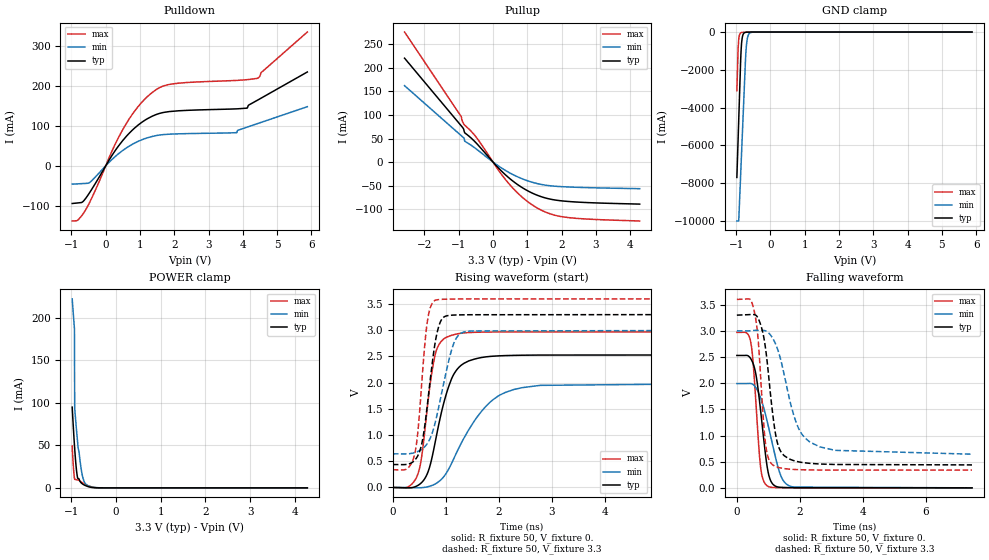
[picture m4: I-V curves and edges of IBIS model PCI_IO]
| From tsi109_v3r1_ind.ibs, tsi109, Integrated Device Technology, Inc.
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|   MODEL PCI_IO
[Model]   PCI_IO
Model_type  I/O
C_comp 4.536p 4.202p 4.874p
Polarity   Non-Inverting
Enable   Active-High
Vinl =   0.80V
Vinh =   2.00V
Vmeas =   1.50V
Cref =   10pF
Rref =   50
Vref=   0.0V
[Model Spec]
[Temperature Range]   27.0   125.0   -40.0
[Voltage Range] 3.3 3. 3.6
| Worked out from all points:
|   slope of the pulldown table from 0 to 0.495 V, typ, clamps not added: 7.81 ohm
|   slope of the pullup table from 0 to 0.495 V, typ, clamps not added: 13.9 ohm
|   GND clamp passes 1 mA (typ) near -0.58 V on its own axis
|   POWER clamp passes 1 mA (typ) near -0.59 V on its own axis
|   rising waveform, R_fixture 50, V_fixture 0.: 20-80 % time 365ps typ, 723ps min, 222ps max; typ from 0 V to 2.53 V
|   rising waveform, R_fixture 50, V_fixture 3.3: 20-80 % time 214ps typ, 317ps min, 159ps max; typ from 0.438 V to 3.3 V
|   falling waveform, R_fixture 50, V_fixture 0.: 20-80 % time 295ps typ, 484ps min, 203ps max; typ from 2.53 V to 0 V
|   falling waveform, R_fixture 50, V_fixture 3.3: 20-80 % time 338ps typ, 623ps min, 226ps max; typ from 3.3 V to 0.438 V
[Pulldown]
-976.9mV  -94.66mA   -46.06mA   -138.7mA
-817.5mV  -93.23mA   -45.29mA   -136.5mA
-595.7mV  -83.14mA   -44.21mA   -112.2mA
-429.3mV  -61.97mA   -39.17mA   -84.92mA
492.7mV   63.11mA    38.33mA    90.31mA
936.3mV   101.8mA    61.1mA     147.9mA
1.352V    124.6mA    73.73mA    184.1mA
1.851V    136.3mA    79.48mA    204.5mA
3.82V     143.1mA    83.35mA    214.6mA
4.125V    144.9mA    97.25mA    216.4mA
4.43V     165.1mA    106.2mA    220mA
5.879V    235.8mA    148.6mA    336.1mA
[Pullup]
-2.579V   220.8mA    162.3mA    276.3mA
-929mV    77.21mA    56.24mA    96.97mA
-887.4mV  73.58mA    53.57mA    85.73mA
-838.9mV  65.18mA    49.35mA    79.56mA
-818.1mV  61.78mA    43.99mA    77.84mA
-471.5mV  38.99mA    26.83mA    51.07mA
277.2mV   -21.28mA   -14.01mA   -29.14mA
623.8mV   -42.97mA   -28.22mA   -58.92mA
942.6mV   -58.4mA    -38.19mA   -80.33mA
1.442V    -74.52mA   -48.11mA   -103.5mA
1.969V    -82.31mA   -52.22mA   -115.7mA
4.277V    -89.5mA    -56.68mA   -125.4mA
[GND Clamp]
-976.9mV  -7.694A    -10A       -3.11A
-940.4mV  -5.645A    -10A       -848.5mA
-923.3mV  -4.682A    -10A       -400.9mA
-899.6mV  -3.359A    -8.991A    -148.3mA
-863.2mV  -1.353A    -7.407A    -43.18mA
-837.4mV  -553.5mA   -6.29A     -25.04mA
-794.5mV  -126.9mA   -4.431A    -15.74mA
-727.9mV  -18.49mA   -1.562A    -9.993mA
-708.6mV  -11.57mA   -935.5mA   -8.672mA
-670mV    -5.111mA   -330.6mA   -6.269mA
-603.5mV  -1.592mA   -60.06mA   -2.971mA
5.879V    0A         0A         0A
[Power Clamp]
-976.9mV  94.83mA    222.1mA    49.21mA
-949.3mV  68.95mA    202.6mA    23.59mA
-927.1mV  50.38mA    187.5mA    11.34mA
-921.6mV  46.09mA    93.87mA    10.01mA
-888.4mV  24.44mA    72.65mA    9.649mA
-855.2mV  11.42mA    53.18mA    9.29mA
-783.3mV  6.267mA    24.59mA    7.167mA
-750.1mV  4.693mA    14.57mA    6.03mA
-705.8mV  3.303mA    6.993mA    4.715mA
-656.1mV  2.103mA    3.495mA    3.408mA
-357.3mV  8.391uA    72.94uA    14.41uA
4.277V    0A         0A         0A
[Ramp]
dV/dt_r 1.518/365.23p 1.196/721.023p 1.782/221.8p
dV/dt_f 1.717/337.435p 1.415/622.991p 1.957/226.082p
[Rising Waveform]
R_fixture = 50
V_fixture = 0.
0s        0V         0V         0V
470ps     37.05mV    -6.726mV   246.6mV
550ps     99.96mV    -3.323mV   620.7mV
650ps     259.3mV    11.36mV    1.507V
800ps     863.9mV    67.25mV    2.539V
1.05ns    1.912V     341.7mV    2.883V
1.27ns    2.315V     802.2mV    2.942V
1.67ns    2.48V      1.449V     2.965V
2.28ns    2.522V     1.869V     2.969V
7.47ns    2.529V     1.993V     2.97V
[Rising Waveform]
R_fixture = 50
V_fixture = 3.3
V_fixture_min = 3.
V_fixture_max = 3.6
0s        438.2mV    642.1mV    338.6mV
410ps     515.4mV    664.5mV    626mV
470ps     601.9mV    685.9mV    1.029V
550ps     848.7mV    731.3mV    2.042V
650ps     1.557V     836.6mV    3.151V
800ps     2.767V     1.238V     3.573V
930ps     3.219V     1.841V     3.591V
1.13ns    3.29V      2.691V     3.596V
1.35ns    3.296V     2.969V     3.599V
7.47ns    3.3V       3V         3.6V
[Falling Waveform]
R_fixture = 50
V_fixture = 0.
0s        2.529V     1.993V     2.97V
440ps     2.469V     1.994V     2.787V
510ps     2.384V     1.976V     2.438V
600ps     2.182V     1.917V     1.677V
760ps     1.445V     1.712V     366.7mV
980ps     340.4mV    1.227V     32.06mV
1.12ns    87.95mV    862.5mV    8.858mV
1.38ns    10.32mV    256.9mV    3.596mV
1.74ns    3.211mV    22.96mV    1.388mV
7.47ns    1.068uV    15.07uV    0V
[Falling Waveform]
R_fixture = 50
V_fixture = 3.3
V_fixture_min = 3.
V_fixture_max = 3.6
0s        3.3V       3V         3.6V
420ps     3.311V     3.001V     3.601V
560ps     3.308V     3.009V     3.356V
680ps     3.232V     3.01V      2.799V
910ps     2.668V     3V         845.2mV
1.15ns    1.357V     2.845V     435.1mV
1.44ns    655.6mV    2.332V     374.1mV
1.88ns    507.9mV    1.256V     349.5mV
2.32ns    467.9mV    874.5mV    342.5mV
7.47ns    438.2mV    643.1mV    338.6mV
